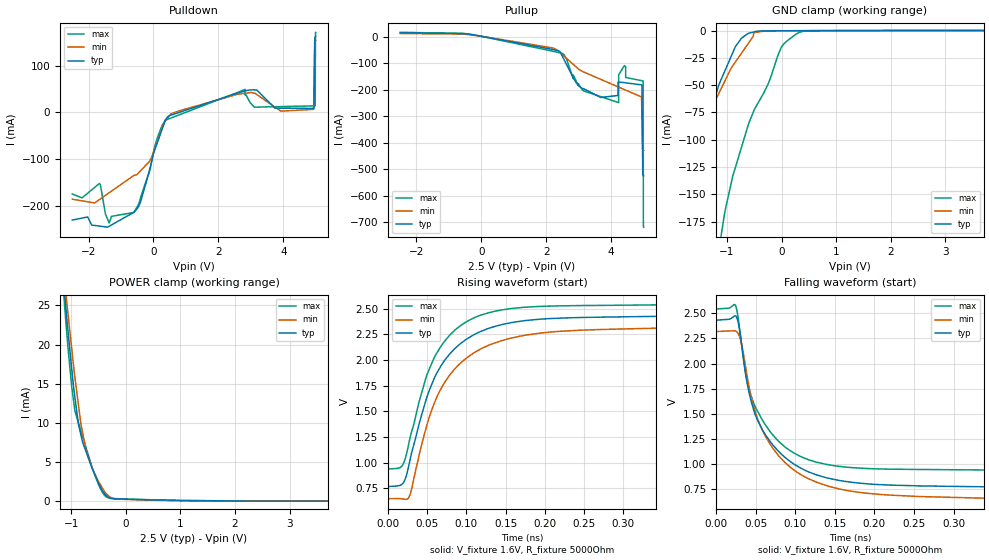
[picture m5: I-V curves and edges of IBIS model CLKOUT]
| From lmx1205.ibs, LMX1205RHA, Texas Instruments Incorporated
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|   Model CLKOUT
[Model]   CLKOUT
Model_type   Output
Polarity   Non-Inverting
Vmeas = 1.25
Vref = 1.25
Cref = 2pF
Rref = 50
|   typ   min   max
C_comp   0.469pF   0.387pF   0.542pF
[Voltage Range]   2.5   2.4   2.6
[Temperature Range]   27   105   -40
[Pullup Reference]   2.5   2.4   2.6
[Pulldown Reference]   -0   0   -0
[Power Clamp Reference]   2.5   2.4   2.6
[GND Clamp Reference]   0   0   0
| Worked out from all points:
|   slope of the pulldown table from 0 to 0.375 V, typ, clamps not added: 5.07 ohm
|   slope of the pullup table from 0 to 0.375 V, typ, clamps not added: 44.5 ohm
|   GND clamp passes 1 mA (typ) near -0.49 V on its own axis
|   POWER clamp passes 1 mA (typ) near -0.39 V on its own axis
|   falling waveform, V_fixture 1.6V, R_fixture 5000Ohm: 20-80 % time 48.4ps typ, 54.7ps min, 43.5ps max; typ from 2.43 V to 0.767 V
|   rising waveform, V_fixture 1.6V, R_fixture 5000Ohm: 20-80 % time 53.3ps typ, 57.7ps min, 47.7ps max; typ from 0.767 V to 2.43 V
[Pulldown]
|   Voltage   I(typ)   I(min)   I(max)
-2.5V     -231mA     -186.2mA   -175mA
-1.665V   -244mA     -187mA     -152.4mA
-1.364V   -244.3mA   -172.3mA   -237.3mA
-601.3mV  -214.1mA   -135.3mA   -214.7mA
486.2mV   -6.968mA   -7.2mA     -13.35mA
2.822V    46.31mA    41.17mA    49.49mA
4.935V    8.962mA    6.621mA    14.16mA
4.946V    8.959mA    55.62mA    14.18mA
4.973V    161mA      152.7mA    14.22mA
4.983V    162mA      153.6mA    14.24mA
4.992V    162.8mA    154.2mA    171.2mA
5V        163.6mA    154.9mA    172.1mA
[GND Clamp]
|   Voltage   I(typ)   I(min)   I(max)
-2.5V     -293.7mA   -228.1mA   -568.5mA
-2.107V   -226.2mA   -175.6mA   -484.3mA
-1.791V   -172.1mA   -133.5mA   -426.4mA
-1.146V   -49.57mA   -57.33mA   -200.9mA
-1.052V   -38.61mA   -47.64mA   -170.2mA
-846.3mV  -14.86mA   -28.91mA   -125.6mA
-609mV    -2.56mA    -11.83mA   -86.27mA
-511.6mV  -1.322mA   -2.035mA   -74.07mA
-247mV    -298.1uA   -424.6uA   -49.04mA
-7.761mV  -249.5uA   -226.8uA   -15.68mA
335.1mV   -181.6uA   -162.3uA   -1.557mA
5V        0A         0A         0A
[Pullup]
|   Voltage   I(typ)   I(min)   I(max)
-2.5V     14.05mA    11.84mA    16.2mA
2.497V    -74.63mA   -68.02mA   -63.7mA
3.684V    -229.7mA   -161.6mA   -226.7mA
4.231V    -171.1mA   -190.5mA   -249.1mA
4.231V    -171.1mA   -190.5mA   -144mA
4.405V    -173.8mA   -199.7mA   -109.3mA
4.935V    -182mA     -227.7mA   -166.1mA
4.946V    -182.1mA   -293.9mA   -166.4mA
4.973V    -520mA     -425.3mA   -167.1mA
4.983V    -522mA     -426.9mA   -167.3mA
4.992V    -523.6mA   -428.2mA   -716.8mA
5V        -525.2mA   -429.5mA   -719mA
[POWER Clamp]
|   Voltage   I(typ)   I(min)   I(max)
-2.5V     149.5mA    134.9mA    166.7mA
-1.288V   40.48mA    40.81mA    40.83mA
-1.101V   25.15mA    26.89mA    23.42mA
-1.081V   23.5mA     25.48mA    21.64mA
-988.5mV  16.94mA    19.5mA     14.63mA
-928.5mV  13.2mA     15.74mA    11.48mA
-862.1mV  9.726mA    12.12mA    9.956mA
-728.2mV  6.361mA    6.53mA     6.888mA
-505.8mV  2.426mA    2.613mA    2.251mA
-361.6mV  752.6uA    989.8uA    561.2uA
1.146V    92.15uA    8.912uA    31.56uA
5V        0A         0A         0A
[Ramp]
R_load = 5000
|   typ   min   max
dV/dt_r   0.998305/5.33202e-11   1.00256/5.76547e-11   0.962531/4.7611e-11
dV/dt_f   0.998524/4.84121e-11   1.00247/5.45893e-11   0.963054/4.34363e-11
[Falling Waveform]
V_fixture = 1.6V
V_fixture_min = 1.481V
V_fixture_max = 1.74V
R_fixture = 5000Ohm
C_fixture = 0F
|   Time   V(typ)   V(min)   V(max)
0s        2.431V     2.319V     2.542V
23ps      2.471V     2.326V     2.588V
26ps      2.463V     2.318V     2.544V
31ps      2.269V     2.235V     2.27V
38ps      1.868V     1.937V     1.872V
49ps      1.504V     1.535V     1.579V
74ps      1.169V     1.133V     1.268V
113ps     935mV      868.2mV    1.054V
208ps     793.6mV    696.1mV    950.1mV
499ps     766.9mV    647.9mV    936.4mV
[Rising Waveform]
V_fixture = 1.6V
V_fixture_min = 1.481V
V_fixture_max = 1.74V
R_fixture = 5000Ohm
C_fixture = 0F
|   Time   V(typ)   V(min)   V(max)
0s        766.9mV    647.3mV    936.9mV
18ps      788.7mV    645.7mV    969.1mV
26ps      953.1mV    652.6mV    1.168V
48ps      1.598V     1.322V     1.816V
63ps      1.882V     1.65V      2.077V
84ps      2.101V     1.903V     2.282V
114ps     2.263V     2.089V     2.425V
157ps     2.364V     2.213V     2.501V
208ps     2.404V     2.273V     2.526V
499ps     2.431V     2.318V     2.541V
